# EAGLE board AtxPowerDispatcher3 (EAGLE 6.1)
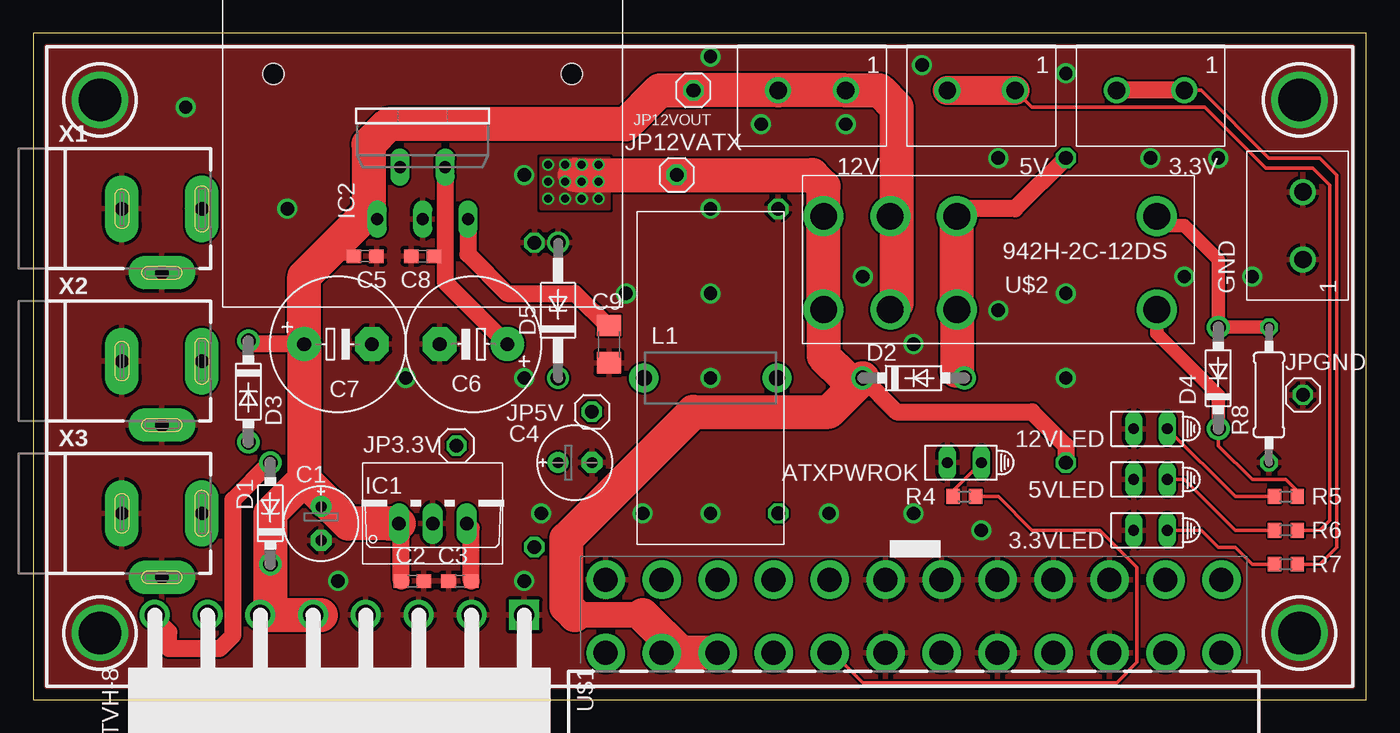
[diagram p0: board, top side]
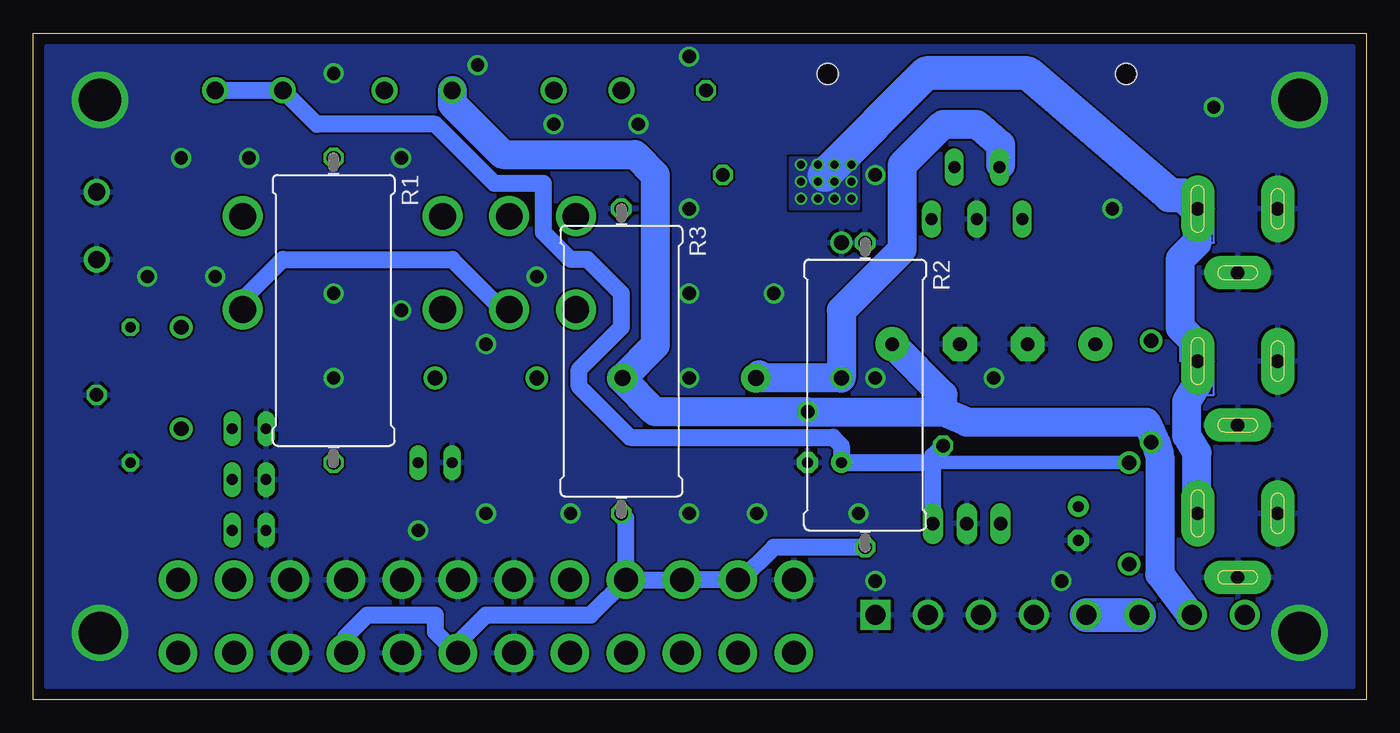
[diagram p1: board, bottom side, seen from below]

Size 100 x 50 mm. Coordinates in mm from the lower left corner, seen from the top.
Outline: 0,0 100,0 100,50 0,50 0,0
Copper layers (1*16): Top 0.035mm / dielectric 1.5mm / Bottom 0.035mm
Design rules: minimum track width 6mil, minimum drill 12mil, track to track 6mil, track to pad 6mil, pad to pad 6mil, via to via 6mil, smd to smd 0mil, copper to edge 0mil, drill to drill 10mil, minimum pad ring 10mil, minimum via ring 6mil, stop-mask expansion 2mil, vias tented up to drill 100mil, thermal gap 10mil

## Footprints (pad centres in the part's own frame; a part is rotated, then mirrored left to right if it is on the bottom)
1X02_BIG = drill 1.3: P$1 0,0; P$2 5.08,0
HLMP6 = drill 0.813 long: A -1.27,0; K 1.27,0
E2,5-6E = drill 0.813 pad 1.575: + -1.27,0 | drill 0.813 pad 1.575 octagon: - 1.27,0
C0603 = smd 1.1 x 1: 1 -0.85,0; 2 0.85,0
E5-10,5 = drill 1.016 pad 2.54: + -2.54,0 | drill 1.016 pad 2.54 octagon: - 2.54,0
C1206 = smd 1.6 x 1.8: 1 -1.4,0; 2 1.4,0
DO41-7.6 = drill 1.1 pad 1.7: A 3.81,0; C -3.81,0
DO41Z10 = drill 1.118: A 5.08,0; C -5.08,0
TO220V = drill 1.016 long: 1 -2.54,-2.54; 2 0,-2.54; 3 2.54,-2.54
TO220-5 = drill 0.9 long: 1 -3.4,-8.4; 2 -1.7,-4.5; 3 0,-8.4; 4 1.7,-4.5; 5 3.4,-8.4 | hole 1.6: -11.2,2.5; 11.2,2.5
ATX24_RIGHT_ANGLE = drill 1.8 pad 2.9: 1 23.1,4.76; 2 18.9,4.76; 3 14.7,4.76; 4 10.5,4.76; 5 6.3,4.76; 6 2.1,4.76; 7 -2.1,4.76; 8 -6.3,4.76; 9 -10.5,4.76; 10 -14.7,4.76; 11 -18.9,4.76; 12 -23.1,4.76; 13 23.1,10.26; 14 18.9,10.26; 15 14.7,10.26; 16 10.5,10.26; 17 6.3,10.26; 18 2.1,10.26; 19 -2.1,10.26; 20 -6.3,10.26; 21 -10.5,10.26; 22 -14.7,10.26; 23 -18.9,10.26; 24 -23.1,10.26
1X01 = drill 1.016 octagon: 1 0,0
2200-12.7 = drill 1.2 pad 2.184: 1 -5,0; 2 5,0
0922/22 = drill 1.016 octagon: 1 -11.43,0; 2 11.43,0
R0603 = smd 1 x 1.1: 1 -0.85,0; 2 0.85,0
0207/10 = drill 0.813 octagon: 1 -5.08,0; 2 5.08,0
VH_8 = drill 1.5 square: 1 0,0 | drill 1.5: 2 3.96,0; 3 7.92,0; 4 11.88,0; 5 15.84,0; 6 19.8,0; 7 23.76,0; 8 27.72,0
942H = drill 2: 1 -11.9,3.75; 2 3.1,3.75; 3 8.1,3.75; 4 13.1,3.75; '1 -11.9,-3.25; '2 3.1,-3.25; '3 8.1,-3.25; '4 13.1,-3.25
2DC-0005D100 = drill 1 pad 2.5 long: 1 3.75,0; 2 -2.25,0; 3 0.75,-4.8

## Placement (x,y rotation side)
3.3V  [1X02_BIG]  86.36,45.72 180 top
3.3VLED  HLMP6  [HLMP6]  83.82,12.7 180 top
5V  [1X02_BIG]  73.66,45.72 180 top
5VLED  HLMP6  [HLMP6]  83.82,16.51 180 top
12V  [1X02_BIG]  60.96,45.72 180 top
12VLED  HLMP6  [HLMP6]  83.82,20.32 180 top
ATXPWROK  HLMP6  [HLMP6]  69.85,17.78 180 top
C1  33u  [E2,5-6E]  21.59,13.21 270 top
C2  0.1u  [C0603]  28.45,8.89 0 top
C3  0.1u  [C0603]  32,8.89 180 top
C4  100u  [E2,5-6E]  40.64,17.78 0 top
C5  0.1u  [C0603]  24.89,33.27 0 top
C6  1000uF low-ESR  [E5-10,5]  22.86,26.67 0 top
C7  1000uF low-ESR  [E5-10,5]  33.02,26.67 180 top
C8  0.1u  [C0603]  29.21,33.27 180 top
C9  10u  [C1206]  43.18,26.67 270 top
D1  1N5817-B  [DO41-7.6]  17.78,13.97 90 top
D2  1N5817-B  [DO41-7.6]  66.04,24.13 0 top
D3  1N5817-B  [DO41-7.6]  16.13,23.11 270 top
D4  1N5817-B  [DO41-7.6]  88.9,24.13 90 top
D5  1N4728  [DO41Z10]  39.37,29.21 90 top
GND  [1X02_BIG]  95.25,33.02 90 top
IC1  788TV  [TO220V]  29.97,15.75 0 top
IC2  SI-8050  [TO220-5]  29.21,44.45 0 top
J1  ATX24RH  [ATX24_RIGHT_ANGLE]  66.04,-1.27 0 top
JP3.3V  [1X01]  31.75,19.05 90 top
JP5V  [1X01]  41.91,21.59 0 top
JP12VATX  [1X01]  48.26,39.37 0 top
JP12VOUT  [1X01]  49.53,45.72 180 top
JPGND  [1X01]  95.25,22.86 0 top
L1  47uH  [2200-12.7]  50.8,24.13 0 top
R1  30 5W  [0922/22]  77.47,29.21 270 bottom
R2  5 5W  [0922/22]  37.59,22.86 270 bottom
R3  5 5W  [0922/22]  55.88,25.4 270 bottom
R4  1k  [R0603]  69.85,15.24 0 top
R5  1k  [R0603]  93.98,15.24 0 top
R6  1k  [R0603]  93.98,12.7 0 top
R7  1k  [R0603]  93.98,10.16 0 top
R8  90ohm 1/4W  [0207/10]  92.71,22.86 90 top
U$1  TUS_POWER_SOCKETVH-8  [VH_8]  36.83,6.35 180 top
U$2  942H-2C-12DS  [942H]  72.39,33.02 180 top
X1  DCJACK  [2DC-0005D100]  8.89,36.83 0 top
X2  DCJACK  [2DC-0005D100]  8.89,25.4 0 top
X3  DCJACK  [2DC-0005D100]  8.89,13.97 0 top

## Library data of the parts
3.3V 5V 12V GND IC1 IC2 L1 U$1 U$2 = myparts
3.3VLED 5VLED 12VLED ATXPWROK = display-hp; MF: AGILENT TECHNOLOGIES; MPN: HLMP-6500; OC_FARNELL: 1652490; OC_NEWARK: 40K0088
C1-C9 R4-R7 = rcl
D1-D5 = diode
J1 = SparkFun
JP3.3V JP5V JP12VATX JP12VOUT JPGND = pinhead
R1-R3 R8 = resistor
X1-X3 = kamiki-dcjack

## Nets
3.3V: 3.3V.P$1 3.3V.P$2 C3.1 C4.+ D1.A IC1.3 JP3.3V.1 R7.2 U$1.8
+5V: 5V.P$1 5V.P$2 C7.+ C8.1 D3.A IC2.4 JP5V.1 L1.2 R6.2 U$1.7
+12V: 12V.P$1 12V.P$2 C1.+ C2.1 C5.1 C6.+ D1.C D3.C D4.C IC1.1 IC2.1 JP12VOUT.1 R5.2 U$1.5 U$1.6 U$2.1 U$2.3 U$2.'3
GND: 3.3VLED.K 5VLED.K 12VLED.K ATXPWROK.K C1.- C2.2 C3.2 C4.- C5.2 C6.- C7.- C8.2 C9.2 D5.A GND.P$1 GND.P$2 IC1.2 IC2.3 J1.3 J1.5 J1.7 J1.15 J1.16 J1.17 J1.18 J1.19 J1.24 JPGND.1 R2.1 R3.1 R8.1 U$1.1 U$1.2 U$1.3 U$1.4 X1.2 X1.3 X2.2 X2.3 X3.2 X3.3
N$1: 12VLED.A R5.1
N$2: J1.8 R4.2
N$3: J1.4 J1.6 J1.21 J1.22 J1.23 R2.2 R3.2
N$4: 5VLED.A R6.1
N$5: 3.3VLED.A R7.1
N$6: ATXPWROK.A R4.1
N$8: D4.A R8.2 U$2.'1
N$9: D5.C IC2.2 L1.1
N$10: D2.A R1.1 U$2.2 U$2.'2
N$11: D2.C J1.10 J1.11 JP12VATX.1 R1.2 U$2.4 U$2.'4 X1.1 X2.1 X3.1
N$17: C9.1 IC2.5

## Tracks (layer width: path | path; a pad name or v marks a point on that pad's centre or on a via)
3.3V
  Top 0.152: 8.89,6.35 U$1.8
  Top 0.254: R7.2 96.52,10.16 97.79,11.43 97.79,39.37 96.52,40.64 92.71,40.64 87.63,45.72 3.3V.P$1
  Top 1.27: 3.3V.P$1 3.3V.P$2 | U$1.8 9.11,6.32 | D1.A 14.99,14.99 14.99,4.83 13.97,3.81 10.16,3.81 10.16,5.08 8.89,6.35 | C3.1 32.85,12.87 IC1.3
  Bottom 1.016: 32.51,17.78 D1.A | IC1.3 32.51,13.46
  Bottom 1.27: 3.3V.P$1 3.3V.P$2 78.74,43.18 69.85,43.18 65.41,38.73 61.72,38.73 61.72,35.05 59.69,33.02 58.42,33.02 55.88,30.48 55.88,27.94 59.05,24.77 59.05,23.5 55.24,19.68 40.01,19.68 39.37,19.05 C4.+ 32.51,17.78 | 32.51,13.46 32.51,17.78 | 32.51,17.78 32.51,18.29 JP3.3V.1
+5V
  Top 0.152: C8.1 30.48,33.02 30.91,33.02
  Top 0.254: 5V.P$1 74.93,44.45 87.88,44.45 92.46,39.88 96.01,39.88 97.28,38.61 97.28,13.46 96.52,12.7 R6.2
  Top 1.27: IC2.4 30.91,33.02 30.91,31.32 C7.+
  Top 2.184: 5V.P$2 5V.P$1
  Bottom 0.152: 13.21,6.35 U$1.7 | D3.A 16.51,19.05 15.88,19.43
  Bottom 1.27: 53.34,26.59 53.34,26.67 55.88,24.13
  Bottom 2.184: 5V.P$2 68.58,44.7 64.77,40.89 54.86,40.89 53.34,39.37 53.34,26.67 | 31.75,21.59 29.97,20.83 16.51,20.83 15.88,19.43 15.49,18.29 15.49,9.4 13.21,6.35 | 53.34,26.59 L1.2 | 31.75,21.59 31.75,22.86 C7.+ | 31.75,21.59 JP5V.1 53.34,21.59 55.88,24.13
+12V
  Top 0.152: 22.23,33.66 22.86,33.02 24.13,33.02 C5.1 | 17.78,6.35 U$1.6
  Top 0.254: R5.2 94.83,15.66 93.98,16.51 91.44,16.51 88.9,19.05 D4.C
  Top 0.61: 18.63,9.31 D1.C
  Top 1.016: U$2.1 84.29,27.47 88.9,22.86 D4.C
  Top 1.27: 24.62,36.05 IC2.1 25.15,36.21 | 64.77,36.75 U$2.'3 | 64.77,29.75 U$2.3 | C6.+ 16.38,26.67 D3.C | 17.78,8.89 18.2,9.31 18.2,9.74 D1.C | C2.1 27.6,12.28 26.67,13.21 | 23.62,13.21 22.86,13.21 C1.+
  Top 2.54: 24.62,36.05 22.23,33.66 20.32,31.75 C6.+ 20.32,16.51 | 25.15,36.21 25.15,41.66 26.67,43.18 44.45,43.18 46.99,45.72 JP12VOUT.1 12V.P$2 12V.P$1 63.5,45.72 64.77,44.45 64.77,36.75 64.77,29.75 | 21.59,6.35 17.78,6.35 17.78,8.89 D1.C 17.78,13.97 20.32,16.51 | 20.32,16.51 23.62,13.21 26.67,13.21 IC1.1
  Bottom 0.152: 64.77,29.21 U$2.3
  Bottom 1.27: U$2.1 84.29,30.01 81.28,33.02 68.58,33.02 64.77,29.21 63.5,29.21
  Bottom 2.54: U$1.5 U$1.6
GND  (via drill 1, 3.2)
  other vias: 5,45 5,5 95,45 95,5 11.43,44.45 19.05,36.83 77.47,46.99 60.96,43.18 50.8,48.26 77.47,30.48 77.47,24.13 71.12,12.7 72.39,29.21 72.39,40.64 66.04,13.97 66.04,26.67 62.23,31.75 66.67,47.62 59.69,13.97 50.8,13.97 50.8,24.13 50.8,30.48 50.8,36.83 54.61,43.18 45.72,13.97 38.1,13.97 36.83,24.13 36.83,39.37 36.83,8.89 83.82,40.64 88.9,40.64 86.36,31.75 91.44,31.75 44.45,30.48 22.86,8.89 27.94,24.13
  pour Bottom (rank 3): 1,49 1,1 99,1 99,49
  pour Top (rank 3): 1,49 1,1 99,1 99,49
N$1
  Top 0.254: R5.1 90.17,15.24 12VLED.A
N$2
  Top 0.152: 71.12,15.24 R4.2
  Top 0.254: J1.8 60.01,3.49 62.23,1.27 81.28,1.27 82.8,2.79 82.8,9.91 80.01,12.7 74.93,12.7 72.39,15.24 71.12,15.24
N$3
  Bottom 0.152: 46.99,8.89 J1.23
  Bottom 1.27: J1.4 76.54,4.74 74.93,6.35 69.85,6.35 69.85,5.08 68.26,3.49 J1.6 68.14,4.25 66.04,6.35 58.18,6.35 J1.21 | J1.21 J1.22 J1.23 | R2.2 44.45,11.43 46.99,8.89 | J1.21 55.54,13.63 R3.2
N$4
  Top 0.254: R6.1 90.17,12.7 86.36,16.51 5VLED.A
N$5
  Top 0.254: 3.3VLED.A 87.63,12.7 88.9,11.43 90.17,11.43 91.44,10.16 R7.1
N$6
  Top 0.254: R4.1 69,15.66 ATXPWROK.A
N$8
  Top 1.016: R8.2 D4.A 88.9,33.02 86.36,35.56 85,35.56 U$2.'1
N$9
  Bottom 0.152: 45.72,24.13 L1.1
  Bottom 1.27: 27.43,40.13 IC2.2
  Bottom 2.184: 27.43,40.13 27.43,41.66 29.21,43.18 31.75,43.18 34.8,40.13 34.8,33.78 39.37,29.21 D5.C 45.72,24.13 | 45.55,24.38 L1.1
N$10
  Top 1.27: 69.29,24.69 D2.A | R1.1 73.66,36.83 68.58,36.83 69.14,36.27 | 69.14,36.27 69.85,35.56 | U$2.'2 69.14,36.27
  Top 2.54: U$2.'2 U$2.2 69.29,24.69
N$11  (via drill 0.6)
  Top 0.152: 11.43,36.83 X1.1 12.7,36.83
  Top 1.27: R1.2 77.47,19.05 74.93,21.59 64.77,21.59 D2.C 60.96,24.13
  Top 1.93: 45.72,6.35 40.64,6.35
  Top 2.54: J1.11 J1.10 48.58,3.49 45.72,6.35 | 40.64,6.35 40.01,6.99 40.01,12.06 49.53,21.59 59.69,21.59 D2.C | 40.64,39.37 JP12VATX.1 58.42,39.37 59.29,38.5 U$2.'4 U$2.4 59.29,25.8 60.96,24.13
  Bottom 0.152: 13.34,26.04 13.97,25.4 13.97,26.67 13.34,27.3 | X2.1 11.43,25.4 11.43,22.86 12.7,22.86 13.46,22.35 | 12.7,34.29 11.43,34.29 11.43,36.83 X1.1
  Bottom 2.184: X3.1 12.7,13.97 12.7,18.54 13.46,19.81 13.46,22.35 12.7,23.62 12.7,26.67 13.34,27.3 13.97,27.94 13.97,33.02 12.7,34.29 12.7,36.83
  Bottom 2.54: 40.64,39.37 33.02,46.99 25.4,46.99 14.73,37.85 13.72,37.85 12.7,36.83
  other vias: 38.61,40.13 39.88,40.13 41.15,40.13 42.42,40.13 38.61,38.86 39.88,38.86 41.15,38.86 42.42,38.86 42.42,37.59 41.15,37.59 39.88,37.59 38.61,37.59
  pour Top: 38.1,40.64 38.1,36.83 43.18,36.83 43.18,40.64
  pour Bottom: 38.1,40.64 38.1,36.83 43.18,36.83 43.18,40.64
N$17
  Top 0.152: 43.18,27.94 C9.1
  Top 1.27: IC2.5 32.61,33.43 35.56,30.48 40.64,30.48 43.18,27.94

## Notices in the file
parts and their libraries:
SparkFun: Licensing: CC v3.0 Share-Alike You are welcome to use this library for commercial purposes.
